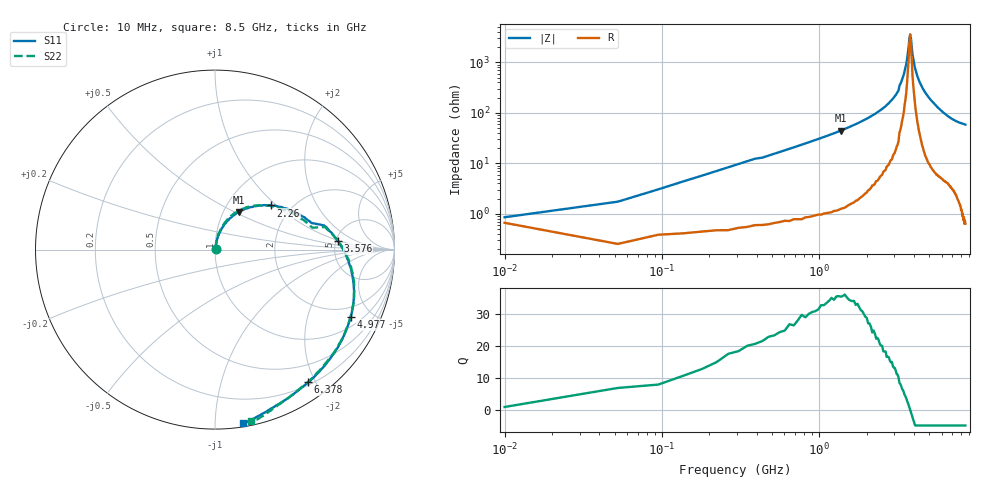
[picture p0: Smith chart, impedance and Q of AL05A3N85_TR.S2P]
!AVX Corporation
!PN: AL05A3N85*TR
!Description: Air Core Inductor, 3.85nH, 4 Turns
!Agilent Technologies,E5071C,MY46102230,A.09.54
!Date: Mon Sep 03 16:08:10 2012
!Data & Calibration Information:
!Freq	S11:SOLT2(ON)	S21:SOLT2(ON)	S12:SOLT2(ON)	S22:SOLT2(ON)
# Hz S dB R 50
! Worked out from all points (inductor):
!   201 points, 10 MHz to 8.5 GHz, reference 50 ohm
!   read as 1/Y11, port 2 shorted: L = 5.07 nH near 52.45 MHz
!   highest Q = 35.7 at 1.368 GHz (marker M1), where L = 5.16 nH
!   self-resonance near 3.746 GHz
!   S11 on the Smith chart (normalised r, x): 10 MHz: 1.01, +0.01; 2.26 GHz: 1.58, +0.92; 3.576 GHz: 5.19, +0.97; 4.977 GHz: 1.44, -3.75; 6.378 GHz: 0.24, -1.90; 8.5 GHz: 0.02, -1.18
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1e7  -46.73 39.8  -0.03 -0.3  -0.14 -0.6  -45.98 39.9
5.245e7  -37.91 73.2  -0.03 -1.2  0.00 -1.3  -37.59 73.9
9.49e7  -33.06 77.3  -0.04 -2.2  -0.03 -2.2  -33.04 77.2
1.3735e8  -29.98 79.1  -0.05 -3.2  -0.03 -3.2  -29.93 78.8
2.2225e8  -25.97 79.2  -0.06 -5.1  -0.04 -5.2  -25.96 79.3
3.496e8  -22.13 77.1  -0.08 -8.0  -0.07 -8.0  -22.10 78.7
7.741e8  -16.55 70.0  -0.17 -17.1  -0.16 -17.2  -16.58 71.0
1.0288e9  -14.28 64.6  -0.26 -22.7  -0.25 -22.8  -14.29 66.0
1.3684e9  -12.07 57.4  -0.40 -30.4  -0.39 -30.5  -12.06 59.5
1.4533e9  -11.58 55.9  -0.44 -32.4  -0.43 -32.4  -11.59 57.2
2.25985e9  -8.02 38.3  -0.97 -51.3  -0.96 -51.4  -8.00 37.4
2.85415e9  -6.02 24.0  -1.53 -65.8  -1.53 -65.8  -6.02 21.5
3.19375e9  -5.09 15.5  -1.93 -74.2  -1.93 -74.2  -5.08 12.6
3.2362e9  -4.13 12.5  -2.48 -76.0  -2.48 -76.0  -4.09 11.7
3.5758e9  -3.27 4.1  -3.16 -83.9  -3.16 -84.0  -3.25 3.9
4.255e9  -2.14 -11.3  -4.61 -99.1  -4.61 -99.2  -2.14 -10.8
4.97665e9  -1.48 -26.3  -6.13 -114.8  -6.13 -114.8  -1.49 -26.2
5.6983e9  -1.11 -41.2  -7.77 -130.5  -7.77 -130.5  -1.12 -42.8
6.3775e9  -0.88 -54.9  -9.68 -144.0  -9.68 -144.0  -0.87 -57.3
7.09915e9  -0.63 -67.2  -12.05 -154.8  -12.05 -154.8  -0.56 -68.5
7.651e9  -0.43 -73.9  -14.01 -160.6  -14.01 -160.7  -0.36 -73.4
8.5e9  -0.17 -80.7  -17.52 -169.9  -17.52 -170.0  -0.20 -78.3
